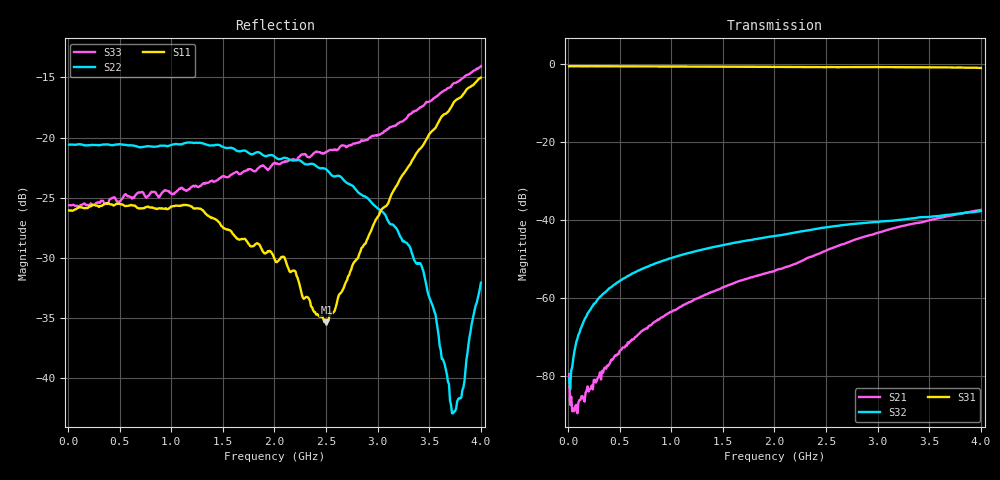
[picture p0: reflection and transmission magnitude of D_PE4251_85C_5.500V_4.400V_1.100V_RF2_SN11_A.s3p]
! Device ID: PE4251_SoldCshunt_081809
! Dir: c:\Test Bench Repositories\Bench_Software_CVI_Version_8\trunk\PSC 4Port_VNA Bench\datalog\4250\TEST\PE4251_SoldCshunt_081809\85C\5p500000\RF2
! Serial: 11
! Insertion: A
! Temp: 85C
! VDD: 5.500
! Control_Hi: 80.000
! Control_Lo: 20.000
! Logic State: RF2
! Port 1: RFC
! Port 2: RF1
! Port 3: RF2
! V1 = 1.10
! V2 = 1.10
! V3 = 1.10
! IDD: 7.018720e-05
! FILE NAME
! DATE 08/18/09  20:19
! CORRECTED  DATA
#  Hz  S  RI  R  50.00
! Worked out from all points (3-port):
!   401 points, 10 MHz to 4 GHz, reference 50 ohm
!   strongest paths, dB at 10 MHz, 1.008 GHz, 2.005 GHz, 3.002 GHz, 4 GHz:
!     S31: -0.6, -0.7, -0.8, -0.8, -1.1
!     S32: -80.6, -49.7, -44.1, -40.5, -37.7
!     S21: -79.5, -63.5, -53.0, -43.3, -37.4
!   lowest |S11| = -35.3 dB at 2.504 GHz (marker M1), VSWR 1.03, Z = 50.4 - j1.67 ohm
!   |S11| at or under -10 dB: start of sweep to end of sweep
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1e7  0.0498 -0.000592  1.78e-05 3.51e-07  0.9307 -0.00301
     0.000105 -7.07e-06  0.0934 -0.000787  7.61e-05 -1.17e-05
     0.9311 -0.00515  2.33e-05 8.99e-05  0.0524 0.00056
1.696e8  0.051 0.000293  9.3e-06 -5.28e-05  0.9292 -0.0597
         1.19e-05 -5.99e-05  0.0929 -0.00372  6.02e-05 0.000576
         0.9295 -0.06  4.7e-05 0.00056  0.0526 0.000252
2.99275e8  0.0515 -0.00118  -4.18e-05 -8.53e-05  0.9244 -0.1061
           -3.24e-05 -9.23e-05  0.0924 -0.00759  7.8e-05 0.000985
           0.9246 -0.1049  8.45e-05 0.000993  0.0535 -0.00282
4.888e8  0.053 -0.00397  -0.000139 -0.000135  0.9125 -0.1694
         -0.000138 -0.000132  0.093 -0.0123  0.000142 0.0016
         0.9131 -0.1684  0.000156 0.00161  0.0538 -0.00557
1.10725e9  0.0506 -0.0127  -0.000792 -0.000144  0.8491 -0.3661
           -0.000782 -0.000145  0.0897 -0.0276  0.000493 0.00355
           0.8505 -0.366  0.000498 0.00355  0.0599 -0.0147
2.005e9  0.0301 -0.00727  -0.00222 -7.6e-05  0.6858 -0.604
         -0.00223 -7.54e-05  0.0767 -0.032  0.00106 0.00614
         0.6864 -0.6039  0.00104 0.00616  0.0686 -0.0383
2.50375e9  0.00442 -0.0165  -0.00405 -0.000364  0.5744 -0.7006
           -0.00406 -0.000384  0.0676 -0.0292  0.00139 0.00792
           0.5761 -0.7012  0.0014 0.00793  0.0501 -0.0715
3.42145e9  -0.082 -0.0388  -0.00908 0.00195  0.3221 -0.8436
           -0.00909 0.00194  0.024 -0.0173  0.00203 0.0106
           0.3257 -0.845  0.00203 0.0107  -0.0359 -0.1288
3.730675e9  -0.1332 -0.0376  -0.011 0.00343  0.2163 -0.8686
            -0.011 0.00342  -0.000356 -0.00715  0.00189 0.0116
            0.2161 -0.8696  0.00188 0.0116  -0.0899 -0.1411
4e9  -0.1749 -0.0298  -0.0125 0.00508  0.1164 -0.8786
     -0.0124 0.00506  -0.0249 -0.00195  0.00199 0.0128
     0.1178 -0.8772  0.00196 0.0128  -0.142 -0.1378
